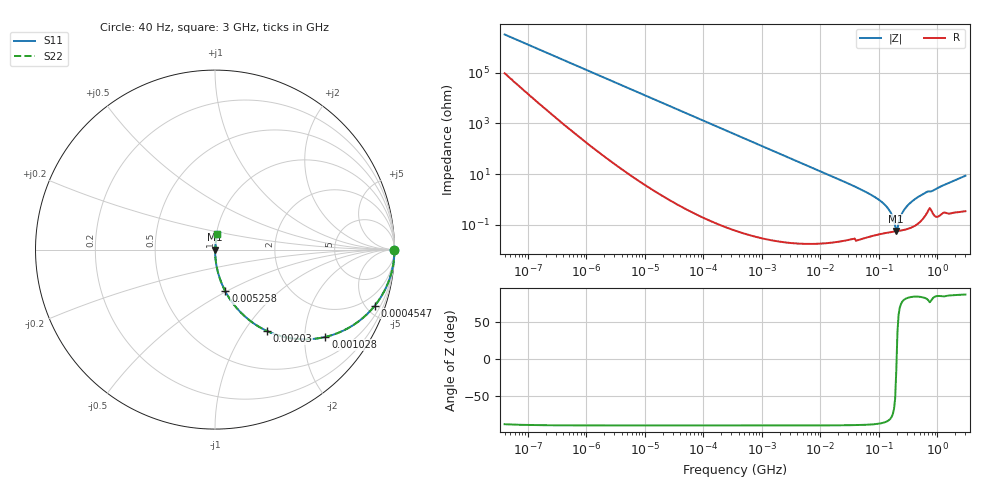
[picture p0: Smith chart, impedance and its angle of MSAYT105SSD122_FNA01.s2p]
! MSAYT105SSD122_FNA01  S-PARAMETER MODEL  ( General Type )
! Model Generated by TAIYO YUDEN Corporation (http://www.ty-top.com)
! Version 2.0
! TAIYO YUDEN Control No. 040624
! Copyright(c) 2004 TAIYO YUDEN CO.,LTD. All Rights Reserved.
! Product Description (link to TY-COMPAS)
! https://ds.yuden.co.jp/TYCOMPAS/or/detail?pn=MSAYT105SSD122KFNA01&u=M
! Products Name : Multilayer Ceramic Capacitors
! Characteristics :
!  Capacitance : 1200 pF , Rated Voltage : 25V
!  Case Size : 1.0 x 0.5 / 0.039 x 0.02 [mm/inch] , Thickness : 0.5 / 0.02 [mm/inch]
!  (Conditions: Temperature = 25 degC , DC Bias Current/Voltage = 0A / 0V)
! External Node Assignments :
!  1  o---| |---o  2
! GND o---------o GND
! Frequency Range : 40Hz  -  3GHz  [ 401 STEP ]
# MHz S RI R 50
! Freq[MHz].  S11 Real  S11 Imag  S21 Real  S21 Imag  S12 Real  S12 Imag  S22 Real  S22 Imag
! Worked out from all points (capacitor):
!   401 points, 40 Hz to 3 GHz, reference 50 ohm
!   read as one part in series: C = 1.23 nF near 44 Hz
!   lowest |Z| = 57.5 mohm at 197.6 MHz (marker M1)
!   series resonance near 200.2 MHz, so ESL is about 520 pH
!   S11 on the Smith chart (normalised r, x): 40 Hz: open; 454.7 kHz: 1.00, -5.71; 1.028 MHz: 1.00, -2.53; 2.03 MHz: 1.00, -1.28; 5.258 MHz: 1.00, -0.49; 3 GHz: 1.01, +0.17
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4e-05  1 -3.08e-05  9.07e-07 3.08e-05  9.07e-07 3.08e-05  1 -3.08e-05
0.000136  1 -0.000105  8.76e-07 0.000105  8.76e-07 0.000105  1 -0.000105
0.000834  1 -0.000642  1.41e-06 0.000642  1.41e-06 0.000642  1 -0.000642
0.017386  0.9998 -0.0134  0.000182 0.0134  0.000182 0.0134  0.9998 -0.0134
0.106589  0.9933 -0.0815  0.0067 0.0815  0.0067 0.0815  0.9933 -0.0815
0.362475  0.9277 -0.2589  0.0723 0.2589  0.0723 0.2589  0.9277 -0.2589
0.454691  0.8908 -0.3118  0.1092 0.3118  0.1092 0.3118  0.8908 -0.3118
1.02824  0.6147 -0.4866  0.3853 0.4866  0.3853 0.4866  0.6147 -0.4866
2.029594  0.2906 -0.4539  0.7094 0.4539  0.7094 0.4539  0.2906 -0.4539
5.258354  0.0576 -0.2326  0.9424 0.2326  0.9424 0.2326  0.0576 -0.2326
7.222098  0.0314 -0.1739  0.9686 0.1739  0.9686 0.1739  0.0314 -0.1739
69.67004  0.000603 -0.0162  0.9994 0.0162  0.9994 0.0162  0.000603 -0.0162
114.7124  0.000503 -0.00751  0.9995 0.00751  0.9995 0.00751  0.000503 -0.00751
150.5692  0.000514 -0.00368  0.9995 0.00368  0.9995 0.00368  0.000514 -0.00368
188.875  0.000544 -0.000744  0.9995 0.000744  0.9995 0.000744  0.000544 -0.000744
197.6342  0.000553 -0.000158  0.9994 0.000158  0.9994 0.000158  0.000553 -0.000158
216.3901  0.000572 0.001  0.9994 -0.001  0.9994 -0.001  0.000572 0.001
247.9136  0.000612 0.00275  0.9994 -0.00275  0.9994 -0.00275  0.000612 0.00275
284.0294  0.000668 0.00456  0.9993 -0.00456  0.9993 -0.00456  0.000668 0.00456
427.1222  0.00108 0.0109  0.9989 -0.0109  0.9989 -0.0109  0.00108 0.0109
642.3046  0.00295 0.019  0.997 -0.019  0.997 -0.019  0.00295 0.019
3000  0.0107 0.0849  0.9893 -0.0849  0.9893 -0.0849  0.0107 0.0849
